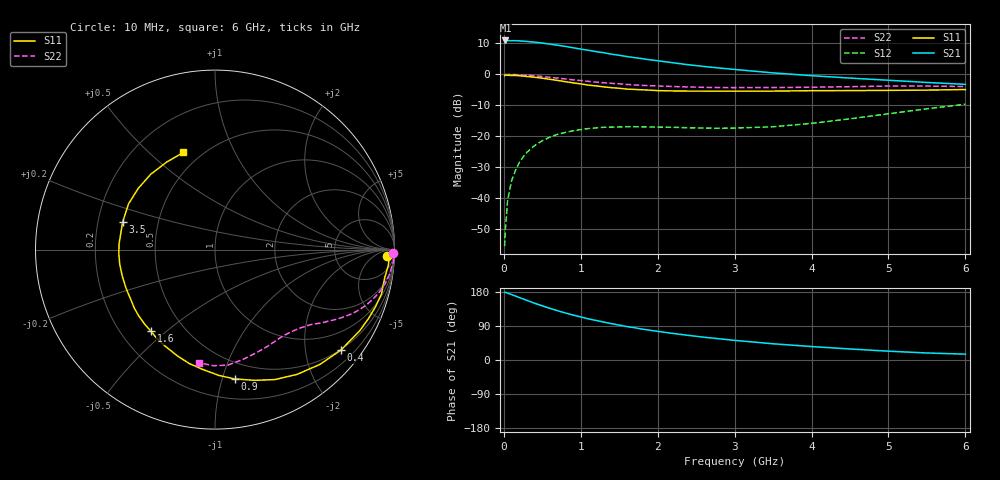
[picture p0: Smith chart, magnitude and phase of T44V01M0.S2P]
! Infineon Technologies  Discrete & RF Semiconductors
! BFR182T
! Si NPN RF Bipolar Junction Transistor in SC75
! VCE = 4 V  IC = 1 mA
! Common Emitter S-Parameters:  October  1999
# GHz  S  MA  R  50
!  f  S11  S21  S12  S22
! GHz  MAG  ANG  MAG  ANG  MAG  ANG  MAG  ANG
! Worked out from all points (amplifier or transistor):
!   36 points, 10 MHz to 6 GHz, reference 50 ohm
!   highest |S21| = 10.9 dB at 20 MHz (marker M1)
!   |S21| within 3 dB of that: start of sweep to 1.055 GHz
!   unconditionally stable (mu >= 1): 2.401 GHz to 4.575 GHz
!   at 250 MHz: K = 0.09, MSG = 18.7 dB, |S12| = -26.7 dB
!   at 1.4 GHz: K = 0.58, MSG = 11.7 dB, |S12| = -17.0 dB
!   at 6 GHz: K = 0.83, MSG = 3.2 dB, |S12| = -9.6 dB
!   S11 on the Smith chart (normalised r, x): 10 MHz: 28, -23; 400 MHz: 0.48, -2.78; 900 MHz: 0.36, -1.10; 1.6 GHz: 0.33, -0.45; 3.5 GHz: 0.31, +0.13; 6 GHz: 0.40, +0.65
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0.01  0.9581 -2.0  3.482 178.7  0.0017 88.3  0.9926 -1.1
0.02  0.9764 -0.7  3.518 178.9  0.0032 97.5  0.989 -0.7
0.05  0.9694 -5.2  3.504 176.3  0.0095 90.2  0.9963 -1.9
0.1  0.9584 -9.5  3.486 172.8  0.0192 86.1  0.9961 -3.8
0.2  0.9493 -19.5  3.465 164.9  0.0377 79.5  0.9844 -7.5
0.3  0.9247 -29.2  3.391 157.4  0.0554 73.1  0.9681 -11.1
0.4  0.8976 -38.6  3.305 149.7  0.0711 67.7  0.946 -14.5
0.5  0.8664 -47.6  3.194 142.9  0.0852 62.4  0.9216 -17.5
0.6  0.8323 -56.6  3.073 136.1  0.0975 57.9  0.896 -20.3
0.7  0.7976 -65.2  2.944 129.9  0.1082 54.1  0.869 -22.8
0.8  0.7618 -73.0  2.823 124.1  0.1161 50.1  0.8426 -25.1
0.9  0.7291 -81.3  2.686 118.6  0.123 46.7  0.8157 -27.1
1.1  0.6713 -95.8  2.444 108.5  0.1338 41.1  0.771 -30.5
1.4  0.6092 -115.6  2.112 95.9  0.1412 34.9  0.7168 -34.8
1.6  0.5782 -128.0  1.936 88.3  0.1433 32.2  0.6876 -37.1
1.8  0.5631 -138.9  1.792 81.5  0.1427 30.6  0.6645 -39.7
2.2  0.5403 -156.6  1.536 70.0  0.1402 30.1  0.6367 -44.3
2.8  0.5363 -177.4  1.266 56.0  0.1352 34.7  0.6123 -52.2
3.5  0.537 163.5  1.056 42.8  0.1429 45.6  0.6133 -61.5
4.5  0.5471 141.5  0.871 29.1  0.192 58.4  0.6324 -76.1
5.5  0.557 119.0  0.74 18.5  0.2787 60.4  0.647 -90.8
6  0.5694 108.0  0.69 15.4  0.3297 57.8  0.6366 -97.8
